[IBIS Ver]   4.1
[File name]   f29h85xzex.ibs
[File Rev]   1.0
[Date]   May 08,2024
[Source]   Cadence SpeedXP Suite XtractIM 18.0.4.05011.160686   004
[Notes]   One-Section RLC
[Disclaimer]   The model given below represents a 204-pin package.
[Copyright]
[Component] f29h85xzex
[Manufacturer] Texas Instruments
[Package]
|   Typ   Min   Max
R_pkg   0.159679576   0.033338   0.27914
L_pkg   3.09171E-09   1.037E-09   6.501E-09
C_pkg   4.79862E-13   3.114E-13   8.045E-13
[Pin]   Signal_name   model_name   R_pin   L_pin   C_pin
A10   GPIO30   BCF3355DSHYPBFZ_USF_7LM   1.45E-01   2.63E-09   3.38E-13
A11   GPIO83   BCF33100DSHYPBFZ_USF_7LM   0.14282   2.63E-09   3.32E-13
A12   GPIO81   BCF33100DSHYPBFZ_USF_7LM   0.14686   2.73E-09   3.47E-13
A13   GPIO77   BCF33100DSHYPBFZ_USF_7LM   0.14855   2.78E-09   4.09E-13
A14   GPIO72   BCF33100DSHYPBFZ_USF_7LM   0.15713   2.98E-09   4.19E-13
A15   GPIO69   BCF33100DSHYPBFZ_USF_7LM   0.14267   2.65E-09   4.90E-13
A2   GPIO13   BCF33100DSHYPBFZ_USF_7LM   1.43E-01   2.73E-09   4.52E-13
A3   GPIO12   BCF33100DSHYPBFZ_CORNER_USF_7LM   1.29E-01   2.21E-09   3.70E-13
A4   GPIO11   BCF33100DSHYPBFZ_USF_7LM   1.39E-01   2.63E-09   3.46E-13
A5   GPIO9   BCF3385DSHYPBFZ_USF_7LM   1.47E-01   2.75E-09   3.42E-13
A6   GPIO5   BCF33100DSHYPBFZ_USF_7LM   1.44E-01   2.67E-09   3.62E-13
A7   GPIO1   BCF33100DSHYPBFZ_USF_7LM   1.23E-01   2.07E-09   3.43E-13
A8   GPIO0   BCF33100DSHYPBFZ_USF_7LM   1.47E-01   2.73E-09   3.11E-13
A9   GPIO29   BQ33100HYPBFZ_PMB_5FS_LC_7LM   1.24E-01   2.04E-09   3.52E-13
B1   GPIO19   BCF33100DSHYPBFZ_USF_7LM   1.48E-01   2.78E-09   4.56E-13
B10   GPIO31   BCF33100DSHYPBFZ_USF_7LM   1.23E-01   2.03E-09   4.04E-13
B11   GPIO85   BCF33100DSHYPBFZ_USF_7LM   0.13246   2.41E-09   3.77E-13
B12   GPIO80   BCF33100DSHYPBFZ_USF_7LM   0.14179   2.59E-09   4.13E-13
B13   GPIO76   BCF33100DSHYPBFZ_USF_7LM   0.14931   2.86E-09   4.41E-13
B14   GPIO71   BCF33100DSHYPBFZ_USF_7LM   0.13499   2.41E-09   4.82E-13
B15   GPIO68   BCF33100DSHYPBFZ_CORNER_USF_7LM   0.12949   2.19E-09   4.03E-13
B16   GPIO67   BCF33100DSHYPBFZ_CORNER_USF_7LM   0.143   2.36E-09   4.11E-13
B2   GPIO17   BCF33100DSHYPBFZ_USF_7LM   1.60E-01   2.91E-09   4.98E-13
B3   GPIO14   BCF33100DSHYPBFZ_CORNER_USF_7LM   1.28E-01   2.08E-09   3.80E-13
B4   GPIO100   BCF33100DSHYPBFZ_USF_7LM   0.11781   2.04E-09   3.20E-13
B5   GPIO101   BCF33100DSHYPBFZ_USF_7LM   0.12464   2.10E-09   3.89E-13
B6   GPIO6   BCF3355DSHYPBFZ_USF_7LM   1.22E-01   2.04E-09   3.60E-13
B7   GPIO2   BCF33100DSHYPBFZ_USF_7LM   1.34E-01   2.44E-09   3.89E-13
B8   GPIO23   BQ33100HYPBFZ_PMB_5FS_LC_7LM   1.41E-01   2.62E-09   3.69E-13
B9   GPIO26   BCF33100DSHYPBFZ_USF_7LM   1.68E-01   3.36E-09   3.87E-13
C1   GPIO20   BCF33100DSHYPBFZ_USF_7LM   1.62E-01   3.26E-09   4.43E-13
C10   GPIO87   BCF33100DSHYPBFZ_USF_7LM   0.12649   2.12E-09   4.99E-13
C11   GPIO86   BCF33100DSHYPBFZ_USF_7LM   0.14552   2.67E-09   4.72E-13
C12   GPIO79   BCF33100DSHYPBFZ_USF_7LM   0.13263   2.32E-09   4.56E-13
C13   GPIO75   BCF33100DSHYPBFZ_USF_7LM   0.14056   2.47E-09   5.63E-13
C14   GPIO70   BCF3385DSHYPBFZ_CORNER_7LM   0.14317   2.50E-09   5.54E-13
C15   GPIO43   BCF33100DSHYPBFZ_CORNER_USF_7LM   0.15632   2.74E-09   4.12E-13
C16   GPIO42   BCPF335585DSHYPBFZ_USF_7LM   0.13495   2.31E-09   3.79E-13
C2   GPIO21   BCF33100DSHYPBFZ_USF_7LM   1.36E-01   2.50E-09   4.05E-13
C3   GPIO88   BCF33100DSHYPBFZ_USF_7LM   0.20709   4.07E-09   5.48E-13
C4   GPIO15   BQ33100HYPBFZ_PMB_5FS_LC_7LM   1.53E-01   2.53E-09   5.23E-13
C5   GPIO10   BQ33100HYPBFZ_PMB_5FS_LC_7LM   1.52E-01   2.77E-09   4.93E-13
C6   GPIO7   BCF33100DSHYPBFZ_USF_7LM   1.41E-01   2.49E-09   4.93E-13
C7   GPIO3   BCF33100DSHYPBFZ_USF_7LM   1.27E-01   2.12E-09   4.77E-13
C8   GPIO24   BCF33100DSHYPBFZ_USF_7LM   1.28E-01   2.12E-09   4.56E-13
C9   GPIO27   BCF33100DSHYPBFZ_USF_7LM   1.53E-01   2.81E-09   4.33E-13
D1   GPIO34   BCF33100DSHYPBFZ_USF_7LM   0.1782   3.51E-09   4.28E-13
D10   GPIO82   BCF33100DSHYPBFZ_USF_7LM   0.19065   3.73E-09   5.54E-13
D11   GPIO84   BCF33100DSHYPBFZ_USF_7LM   0.16159   2.88E-09   5.13E-13
D12   GPIO78   BCF33100DSHYPBFZ_USF_7LM   0.16009   3.23E-09   5.81E-13
D13   GPIO74   BCF33100DSHYPBFZ_USF_7LM   0.15949   3.19E-09   5.75E-13
D14   GPIO46   BCF33100DSHYPBFZ_USF_7LM   0.12327   1.89E-09   4.41E-13
D15   GPIO47   BCF33100DSHYPBFZ_USF_7LM   0.14294   2.62E-09   3.89E-13
D16   GPIO103   BCF33100DSHYPBFZ_USF_7LM   0.12938   2.13E-09   3.83E-13
D2   GPIO91   BCF33100DSHYPBFZ_USF_7LM   0.15495   2.87E-09   4.60E-13
D3   GPIO90   BCF33100DSHYPBFZ_USF_7LM   0.20167   3.98E-09   6.00E-13
D4   GPIO89   BCF33100DSHYPBFZ_USF_7LM   0.18558   3.67E-09   6.22E-13
D5   GPIO16   BCF33100DSHYPBFZ_USF_7LM   1.61E-01   2.51E-09   6.08E-13
D6   GPIO8   BCF33100DSHYPBFZ_USF_7LM   1.54E-01   2.98E-09   4.51E-13
D7   GPIO4   BCF33100DSHYPBFZ_USF_7LM   1.54E-01   2.71E-09   5.71E-13
D8   GPIO25   BCF33100DSHYPBFZ_USF_7LM   1.67E-01   3.27E-09   5.93E-13
D9   GPIO28   BCF33100DSHYPBFZ_USF_7LM   1.54E-01   2.72E-09   4.57E-13
E1   GPIO35   BCF33100DSHYPBFZ_USF_7LM   0.16952   3.23E-09   3.78E-13
E13   GPIO73   BCF33100DSHYPBFZ_USF_7LM   0.17483   3.52E-09   6.78E-13
E14   GPIO38   BCF33100DSHYPBFZ_USF_7LM   0.1436   2.49E-09   5.26E-13
E16   GPIO220,X1   BCPF335585DSHYPBFZ_USF_7LM   4.92E-02   1.43E-09   4.41E-13
E2   GPIO92   BCF3385DSHYPBFZ_USF_7LM   0.17361   3.35E-09   4.10E-13
E3   GPIO93   BCF33100DSHYPBFZ_USF_7LM   0.15008   2.68E-09   4.68E-13
E4   GPIO94   BCF33100DSHYPBFZ_USF_7LM   0.25902   5.43E-09   5.57E-13
E5   GPIO95   BCF33100DSHYPBFZ_USF_7LM   0.23782   5.10E-09   6.10E-13
F1   GPIO22   BQ33100HYPBFZ_PMB_5FS_LC_7LM   1.75E-01   3.52E-09   3.82E-13
F13   GPIO127   BCF33100DSHYPBFZ_USF_7LM   0.15682   3.16E-09   4.43E-13
F14   XRSn   BQ0491FS_3X2_USF_7LM   0.14283   2.45E-09   5.00E-13
F16   GPIO221,X2   BCPF335585DSHYPBFZ_USF_7LM   0.060019   1.35E-09   3.84E-13
F2   GPIO18   BQ33100HYPBFZ_PMB_5FS_LC_7LM   1.76E-01   3.43E-09   4.62E-13
F3   GPIO96   BCF33100DSHYPBFZ_USF_7LM   0.1653   3.12E-09   4.62E-13
F4   GPIO97   BCF33100DSHYPBFZ_USF_7LM   0.19143   3.93E-09   6.19E-13
F5   GPIO98   BCF33100DSHYPBFZ_USF_7LM   0.20928   4.00E-09   6.33E-13
G1   B11,GPIO235   BCF33100DSHYPBFZ_USF_7LM   1.58E-01   3.02E-09   3.27E-13
G13   GPIO66   BCF33100DSHYPBFZ_USF_7LM   0.17577   3.33E-09   5.59E-13
G14   GPIO44   BCF33100DSHYPBFZ_USF_7LM   0.14145   2.56E-09   4.00E-13
G15   GPIO45   BCF33100DSHYPBFZ_USF_7LM   0.13281   2.30E-09   3.62E-13
G16   GPIO32   BCF33100DSHYPBFZ_USF_7LM   1.40E-01   2.46E-09   3.27E-13
G2   B10,GPIO234   BCF33100DSHYPBFZ_USF_7LM   1.52E-01   2.90E-09   4.01E-13
G3   A10,GPIO228   BCF33100DSHYPBFZ_USF_7LM   1.56E-01   3.00E-09   4.95E-13
G4   A11,GPIO229   BCF33100DSHYPBFZ_USF_7LM   1.91E-01   3.93E-09   5.95E-13
G5   GPIO99   BCF33100DSHYPBFZ_USF_7LM   0.21088   4.13E-09   6.03E-13
H1   B9,GPIO233   BCF33100DSHYPBFZ_USF_7LM   1.62E-01   3.18E-09   4.59E-13
H13   GPIO62   BCF33100DSHYPBFZ_USF_7LM   0.17342   3.46E-09   5.40E-13
H14   GPIO63   BCF33100DSHYPBFZ_USF_7LM   0.13389   2.43E-09   4.22E-13
H15   GPIO64   BCF3385DSHYPBFZ_USF_7LM   0.13166   2.33E-09   3.69E-13
H16   GPIO65   BCF33100DSHYPBFZ_USF_7LM   0.14461   2.64E-09   3.20E-13
H2   B8,GPIO232   BCF33100DSHYPBFZ_USF_7LM   1.49E-01   2.88E-09   4.86E-13
H3   A9,GPIO227   BCF33100DSHYPBFZ_USF_7LM   1.52E-01   2.88E-09   4.89E-13
H4   A8,GPIO226   BCF33100DSHYPBFZ_USF_7LM   1.69E-01   3.47E-09   5.54E-13
H5   B7/E27,GPIO231   BCF33100DSHYPBFZ_USF_7LM   1.93E-01   3.96E-09   6.76E-13
J1   B13   ICF33SHYPB_LC_7LM   1.53E-01   3.05E-09   4.14E-13
J13   GPIO61   BCF33100DSHYPBFZ_USF_7LM   0.16898   3.19E-09   4.89E-13
J14   GPIO105   BCF33100DSHYPBFZ_USF_7LM   0.12843   2.17E-09   3.88E-13
J15   GPIO60   BCF33100DSHYPBFZ_USF_7LM   0.13505   2.37E-09   3.84E-13
J16   GPIO59   BCF3385DSHYPBFZ_USF_7LM   0.14954   2.75E-09   3.42E-13
J2   B12   ICF33SHYPB_LC_7LM   1.50E-01   2.94E-09   3.96E-13
J3   B17   ICF33SHYPB_LC_7LM   1.41E-01   2.71E-09   4.68E-13
J4   B16   ICF33SHYPB_LC_7LM   1.75E-01   3.37E-09   6.42E-13
J5   B6/E26,GPIO230   BCF33100DSHYPBFZ_USF_7LM   1.78E-01   3.63E-09   6.64E-13
K1   A13   ICF33SHYPB_LC_7LM   1.32E-01   2.41E-09   3.86E-13
K13   GPIO55   BCF33100DSHYPBFZ_USF_7LM   0.17624   3.49E-09   5.71E-13
K14   GPIO56   BCF33100DSHYPBFZ_USF_7LM   0.14006   2.55E-09   4.56E-13
K15   GPIO57   BCF33100DSHYPBFZ_USF_7LM   0.13532   2.34E-09   3.38E-13
K16   GPIO58   BCF33100DSHYPBFZ_USF_7LM   0.14501   2.61E-09   3.15E-13
K2   A12   ICF33SHYPB_LC_7LM   1.35E-01   2.48E-09   4.10E-13
K3   B5/D31   ICF33SHYPB_LC_7LM   1.61E-01   3.11E-09   4.97E-13
K4   B4/D30   ICF33SHYPB_LC_7LM   1.88E-01   3.80E-09   5.97E-13
K5   A7/E25,GPIO225   BCF33100DSHYPBFZ_USF_7LM   1.67E-01   3.46E-09   6.05E-13
L1   A5/D29   ICF33SHYPB_LC_7LM   1.53E-01   2.89E-09   3.51E-13
L14   GPIO52   BCF33100DSHYPBFZ_USF_7LM   0.16407   3.19E-09   4.14E-13
L15   GPIO53   BCF33100DSHYPBFZ_USF_7LM   0.14307   2.67E-09   3.58E-13
L16   GPIO54   BCF33100DSHYPBFZ_USF_7LM   0.15266   2.85E-09   3.17E-13
L2   A4/D28   ICF33SHYPB_LC_7LM   1.51E-01   2.87E-09   3.95E-13
L3   B3/D27   ICF33SHYPB_LC_7LM   1.10E-01   2.16E-09   4.65E-13
L4   B2/D26   ICF33SHYPB_LC_7LM   1.19E-01   2.52E-09   4.84E-13
L5   A6/E24,GPIO224   BCF33100DSHYPBFZ_USF_7LM   1.86E-01   4.00E-09   5.82E-13
M1   A2/D24   ICF33SHYPB_LC_7LM   1.82E-01   3.69E-09   4.08E-13
M12   FLT3   NC   1.67E-01   3.57E-09   5.24E-13
M13   GPIO51   BCF33100DSHYPBFZ_USF_7LM   0.14778   2.76E-09   5.58E-13
M14   GPIO50   BCF33100DSHYPBFZ_USF_7LM   0.12773   2.25E-09   4.32E-13
M15   GPIO49   BCF33100DSHYPBFZ_USF_7LM   0.1387   2.54E-09   3.84E-13
M16   GPIO219/ERRORSTS   BCF33100DSHYPBFZ_CORNER_USF_7LM   1.51E-01   2.78E-09   3.19E-13
M2   A3/D25   ICF33SHYPB_LC_7LM   1.49E-01   2.79E-09   3.98E-13
M3   A14/B14/C14/D14/E14   ICF33SHYPB_LC_7LM   1.86E-01   3.63E-09   4.91E-13
M4   A15/B15/C15/D15/E15   ICF33SHYPB_LC_7LM   1.93E-01   4.05E-09   5.10E-13
M5   C3/E31   ICF33SHYPB_LC_7LM   1.86E-01   3.93E-09   7.70E-13
M6   D13   ICF33SHYPB_LC_7LM   1.78E-01   3.72E-09   5.83E-13
M7   D12   ICF33SHYPB_LC_7LM   2.03E-01   4.33E-09   6.13E-13
M8   C6,GPIO236   BCF33100DSHYPBFZ_USF_7LM   1.95E-01   4.01E-09   6.43E-13
M9   C7,GPIO237   BCF33100DSHYPBFZ_USF_7LM   1.88E-01   3.84E-09   5.77E-13
N1   VREFLOAB   NC   0.066124   1.95E-09   4.25E-13
N10   D4/B28,GPIO240   BCF33100DSHYPBFZ_USF_7LM   1.99E-01   4.23E-09   6.21E-13
N11   D5/B29,GPIO241   BCF33100DSHYPBFZ_USF_7LM   2.06E-01   4.64E-09   6.26E-13
N12   C8,GPIO238   BCF33100DSHYPBFZ_USF_7LM   2.73E-01   6.23E-09   7.41E-13
N13   E7/A31,GPIO249   BCF33100DSHYPBFZ_USF_7LM   2.30E-01   4.92E-09   7.59E-13
N14   GPIO36   BCF33100DSHYPBFZ_7LM   0.19862   3.66E-09   7.25E-13
N15   GPIO41   BCF33100DSHYPBFZ_CORNER_USF_7LM   0.14183   2.56E-09   3.74E-13
N16   GPIO48   BCF33100DSHYPBFZ_USF_7LM   0.1406   2.41E-09   3.31E-13
N2   VREFHIAB   NC   0.055738   1.97E-09   4.95E-13
N3   B1/C27   ICF33SHYPB_LC_7LM   1.75E-01   3.32E-09   4.83E-13
N4   C2/E30   ICF33SHYPB_LC_7LM   1.76E-01   3.65E-09   7.61E-13
N5   C5   ICF33SHYPB_LC_7LM   9.28E-02   1.96E-09   7.28E-13
N6   D10   ICF33SHYPB_LC_7LM   1.77E-01   3.51E-09   5.14E-13
N7   C16   ICF33SHYPB_LC_7LM   1.71E-01   3.49E-09   5.62E-13
N8   C10   ICF33SHYPB_LC_7LM   1.92E-01   4.15E-09   6.12E-13
N9   E13   ICF33SHYPB_LC_7LM   2.66E-01   6.15E-09   7.62E-13
P1   A1/C25   ICF33SHYPB_LC_7LM   1.71E-01   3.07E-09   3.92E-13
P10   E16   ICF33SHYPB_LC_7LM   1.79E-01   3.54E-09   5.07E-13
P11   E4/A28,GPIO246   BCF33100DSHYPBFZ_USF_7LM   1.88E-01   3.79E-09   5.25E-13
P12   C9,GPIO239   BCF33100DSHYPBFZ_USF_7LM   2.26E-01   5.03E-09   6.33E-13
P13   E6/A30,GPIO248   BCF33100DSHYPBFZ_USF_7LM   1.97E-01   3.93E-09   7.36E-13
P14   GPIO33   BCF33100DSHYPBFZ_7LM   0.18528   3.48E-09   5.63E-13
P15   GPIO39   BCF33100DSHYPBFZ_7LM   0.2243   4.33E-09   4.91E-13
P16   GPIO40   BCF33100DSHYPBFZ_7LM   0.16459   3.13E-09   4.64E-13
P2   B0/C26/VDAC   ICF33SHYPB_LC_7LM   1.78E-01   3.30E-09   4.66E-13
P3   E0/A24/DACC_OUT   ICF33SHYPB_LC_7LM   1.38E-01   2.43E-09   5.71E-13
P4   E1/A25   ICF33SHYPB_LC_7LM   1.35E-01   2.38E-09   6.11E-13
P5   C4   ICF33SHYPB_LC_7LM   8.63E-02   1.54E-09   7.18E-13
P6   D11   ICF33SHYPB_LC_7LM   2.14E-01   4.78E-09   6.22E-13
P7   C17   ICF33SHYPB_LC_7LM   2.12E-01   4.70E-09   6.01E-13
P8   C11   ICF33SHYPB_LC_7LM   1.96E-01   4.14E-09   5.94E-13
P9   E12   ICF33SHYPB_LC_7LM   2.79E-01   6.50E-09   8.05E-13
R1   A0/C24/DACA_OUT   ICF33SHYPB_LC_7LM   1.91E-01   3.62E-09   3.84E-13
R10   E10   ICF33SHYPB_LC_7LM   2.15E-01   4.60E-09   5.82E-13
R11   E5/A29,GPIO247   BCF33100DSHYPBFZ_USF_7LM   1.67E-01   3.21E-09   5.05E-13
R12   D7/B31,GPIO243   BCF33100DSHYPBFZ_USF_7LM   2.16E-01   4.58E-09   5.28E-13
R13   D8/C28,GPIO244   BCF33100DSHYPBFZ_USF_7LM   2.32E-01   4.96E-09   5.66E-13
R14   GPIO223/TDO   BCPF335585DSHYPBFZ_USF_7LM   0.20498   4.09E-09   5.17E-13
R15   TCK   IQ0442FS_40P60P_3X2_USF_7LM   0.20021   3.98E-09   5.32E-13
R16   GPIO37   BCF33100DSHYPBFZ_7LM   0.20499   4.11E-09   4.81E-13
R2   C0/E28   ICF33SHYPB_LC_7LM   1.62E-01   2.97E-09   4.04E-13
R3   D0/B24   ICF33SHYPB_LC_7LM   1.52E-01   2.77E-09   5.12E-13
R4   VREFHICDE   NC   0.033338   1.04E-09   3.47E-13
R5   D2/B26   ICF33SHYPB_LC_7LM   1.38E-01   2.57E-09   3.55E-13
R6   D3/B27   ICF33SHYPB_LC_7LM   1.30E-01   2.35E-09   3.54E-13
R7   D16   ICF33SHYPB_LC_7LM   1.38E-01   2.57E-09   3.57E-13
R8   C12   ICF33SHYPB_LC_7LM   1.31E-01   2.29E-09   3.98E-13
R9   E11   ICF33SHYPB_LC_7LM   1.80E-01   3.64E-09   5.59E-13
T10   E8/C30   ICF33SHYPB_LC_7LM   1.78E-01   3.62E-09   4.04E-13
T11   E17   ICF33SHYPB_LC_7LM   2.17E-01   4.54E-09   5.56E-13
T12   D6/B30,GPIO242   BCF33100DSHYPBFZ_USF_7LM   1.78E-01   3.46E-09   4.08E-13
T13   D9/C29,GPIO245   BCF33100DSHYPBFZ_USF_7LM   1.79E-01   3.36E-09   5.62E-13
T14   GPIO222/TDI   BCF33100DSHYPBFZ_USF_7LM   0.22961   4.78E-09   5.48E-13
T15   TMS   BCF3355DSHYPBFZ_TMS_USF_7LM   0.20987   4.29E-09   5.16E-13
T2   C1/E29   ICF33SHYPB_LC_7LM   1.72E-01   3.35E-09   4.89E-13
T3   D1/B25   ICF33SHYPB_LC_7LM   1.41E-01   2.46E-09   5.13E-13
T4   VREFLOCDE   NC   0.058365   1.77E-09   3.21E-13
T5   E2/A26   ICF33SHYPB_LC_7LM   1.37E-01   2.50E-09   3.26E-13
T6   E3/A27   ICF33SHYPB_LC_7LM   1.26E-01   2.16E-09   3.18E-13
T7   D17   ICF33SHYPB_LC_7LM   1.41E-01   2.60E-09   3.34E-13
T8   C13   ICF33SHYPB_LC_7LM   1.42E-01   2.59E-09   3.52E-13
T9   E9/C31   ICF33SHYPB_LC_7LM   1.55E-01   2.93E-09   3.80E-13
| End of package information
|   Component BCF33100DSHYPBFZ_7LM
[Component]   BCF33100DSHYPBFZ_7LM
[Manufacturer]  IO Methodology Inc.
[Package]
|   typ   min   max
R_pkg   0   0   0
L_pkg   0   0   0
C_pkg   0   0   0
[Pin]   signal_name  model_name   R_pin   L_pin   C_pin
VSS   VSS   GND
VDDS   VDDS   POWER
PAD   PAD   BCF33100DSHYPBFZ_7LM
[Model Selector] BCF33100DSHYPBFZ_7LM
WK_PU_ON_3P3  Cell operated at 3.3(nom)
|WK_PU_ON_3P3; WEAK_PULLUP_ON
WK_PD_ON_3P3  Cell operated at 3.3(nom)
|WK_PD_ON_3P3; WEAK_PULLDOWN_ON
DRIVER_MODE_3P3  Cell operated at 3.3(nom)
|DRIVER_MODE_3P3
RECEIVER_MODE_3P3  Cell operated at 3.3(nom)
|   Component BCF33100DSHYPBFZ_USF_7LM
[Component]   BCF33100DSHYPBFZ_USF_7LM
[Manufacturer]  Texas Instruments
[Package]
| variable   typ   min   max
R_pkg   0.0   0.0   0.0
L_pkg   0.0H   0.0H   0.0H
C_pkg   0.0F   0.0F   0.0F
[Pin]  signal_name   model_name   R_pin   L_pin   C_pin
PAD   PAD   BCF33100_USF_7LM_IO_3.3V   0   0   0
VDDS   VDDS   Power   0   0   0
VSS   VSS   Gnd   0   0   0
[Model Selector] BCF33100DSHYPBFZ_USF_7LM
BCF33100_USF_7LM_IO_3.3V I/O model with 3.3V supply
|   Component BCF33100DSHYPBFZ_CORNER_USF_7LM
[Component]   BCF33100DSHYPBFZ_CORNER_USF_7LM
[Manufacturer]  Texas Instruments
[Package]
| variable   typ   min   max
R_pkg   0.0   0.0   0.0
L_pkg   0.0H   0.0H   0.0H
C_pkg   0.0F   0.0F   0.0F
[Pin]  signal_name   model_name   R_pin   L_pin   C_pin
PAD   PAD   BCF33100_CORNER_7LM_IO_3.3V   0   0   0
VDDS   VDDS   Power   0   0   0
VSS   VSS   Gnd   0   0   0
[Model Selector] BCF33100DSHYPBFZ_CORNER_USF_7LM
BCF33100_CORNER_7LM_IO_3.3V  I/O model with 3.3V supply
|   Component BCF3355DSHYPBFZ_TMS_USF_7LM
[Component]   BCF3355DSHYPBFZ_TMS_USF_7LM
[Manufacturer]  Texas Instruments
[Package]
| variable   typ   min   max
R_pkg   0.0   0.0   0.0
L_pkg   0.0H   0.0H   0.0H
C_pkg   0.0F   0.0F   0.0F
[Pin]  signal_name   model_name   R_pin   L_pin   C_pin
PAD   PAD   BCF3355_TMS_7LM_IO_3.3V   0   0   0
VDDS   VDDS   Power   0   0   0
VSS   VSS   Gnd   0   0   0
[Model Selector] BCF3355DSHYPBFZ_TMS_USF_7LM
BCF3355_TMS_7LM_IO_3.3V I/O model with 3.3V supply
|   Component IQ0442FS_40P60P_3X2_USF_7LM
[Component]   IQ0442FS_40P60P_3X2_USF_7LM
[Manufacturer]  Texas Instruments
[Package]
| variable   typ   min   max
R_pkg   0.0   0.0   0.0
L_pkg   0.0H   0.0H   0.0H
C_pkg   0.0F   0.0F   0.0F
[Pin]  signal_name   model_name   R_pin   L_pin   C_pin
PAD   PAD   IQRX_3.3V   0   0   0
VDDS   VDDS   Power   0   0   0
VSS   VSS   Gnd   0   0   0
[Model Selector] IQ0442FS_40P60P_3X2_USF_7LM
IQRX_3.3V I/O model with 3.3V supply
|   Component BCF3355DSHYPBFZ_USF_7LM
[Component]   BCF3355DSHYPBFZ_USF_7LM
[Manufacturer]  Texas Instruments
[Package]
| variable   typ   min   max
R_pkg   0.0   0.0   0.0
L_pkg   0.0H   0.0H   0.0H
C_pkg   0.0F   0.0F   0.0F
[Pin]  signal_name   model_name   R_pin   L_pin   C_pin
PAD   PAD   BCF3355_USF_7LM_IO_3.3V   0   0   0
VDDS   VDDS   Power   0   0   0
VSS   VSS   Gnd   0   0   0
[Model Selector] BCF3355DSHYPBFZ_USF_7LM
BCF3355_USF_7LM_IO_3.3V I/O model with 3.3V supply
|   Component BCF3385DSHYPBFZ_CORNER_7LM
[Component]   BCF3385DSHYPBFZ_CORNER_7LM
[Manufacturer]  IO Methodology Inc.
[Package]
|   typ   min   max
R_pkg   0   0   0
L_pkg   0   0   0
C_pkg   0   0   0
[Pin]   signal_name  model_name   R_pin   L_pin   C_pin
VSS   VSS   GND
VDDS   VDDS   POWER
PAD   PAD   BCF3385DSHYPBFZ_CORNER_7LM
[Model Selector] BCF3385DSHYPBFZ_CORNER_7LM
WK_PU_ON_3P3_BCF3385DSHYPBFZ_CORNER_7LM  Cell operated at 3.3(nom)
|WK_PU_ON_3P3; WEAK_PULLUP_ON
WK_PD_ON_3P3_BCF3385DSHYPBFZ_CORNER_7LM  Cell operated at 3.3(nom)
|WK_PD_ON_3P3; WEAK_PULLDOWN_ON
DRIVER_MODE_3P3_BCF3385_CORNER_7LM Cell operated at 3.3(nom)
|DRIVER_MODE_3P3
RECEIVER_MODE_3P3_BCF3385_CORNER_7LM  Cell operated at 3.3(nom)
|   Component BCF3385DSHYPBFZ_USF_7LM
[Component]   BCF3385DSHYPBFZ_USF_7LM
[Manufacturer]  Texas Instruments
[Package]
| variable   typ   min   max
R_pkg   0.0   0.0   0.0
L_pkg   0.0H   0.0H   0.0H
C_pkg   0.0F   0.0F   0.0F
[Pin]  signal_name   model_name   R_pin   L_pin   C_pin
PAD   PAD   BCF3385_USF_7LM_IO_3.3V   0   0   0
VDDS   VDDS   Power   0   0   0
VSS   VSS   Gnd   0   0   0
[Model Selector] BCF3385DSHYPBFZ_USF_7LM
BCF3385_USF_7LM_IO_3.3V I/O model with 3.3V supply
|   Component BCPF335585DSHYPBFZ_USF_7LM
[Component]   BCPF335585DSHYPBFZ_USF_7LM
[Manufacturer]  Texas Instruments
[Package]
| variable   typ   min   max
R_pkg   0.0   0.0   0.0
L_pkg   0.0H   0.0H   0.0H
C_pkg   0.0F   0.0F   0.0F
[Pin]  signal_name   model_name   R_pin   L_pin   C_pin
PAD   PAD   BCPF335585DSHYPBFZ_USF_7LM   0   0   0
VDDS   VDDS   Power   0   0   0
VSS   VSS   Gnd   0   0   0
[Model Selector]   BCPF335585DSHYPBFZ_USF_7LM
BCPF335585_7LM_IO_DS0_3.3V   I/O model DS 0 with 3.3V supply
BCPF335585_7LM_IO_DS1_3.3V   I/O model DS 1 with 3.3V supply
|   Component BQ0491FS_3X2_USF_7LM
[Component]   BQ0491FS_3X2_USF_7LM
[Manufacturer]  Texas Instruments
[Package]
| variable   typ   min   max
R_pkg   0.0   0.0   0.0
L_pkg   0.0H   0.0H   0.0H
C_pkg   0.0F   0.0F   0.0F
[Pin]  signal_name   model_name   R_pin   L_pin   C_pin
PAD   PAD   BQ0491FS_3X2_USF_7LM   0   0   0
VDDS   VDDS   Power   0   0   0
VSS   VSS   Gnd   0   0   0
[Model Selector]   BQ0491FS_3X2_USF_7LM
BQ0491_3X2_USF_7LM_IO_15p_3p3   I/O open drain model with C_fixture 15pF for 3.3V supply
BQ0491_3X2_USF_7LM_IO_50p_3p3   I/O open drain model with C_fixture 50pF for 3.3V supply
BQ0491_3X2_USF_7LM_IO_100p_3p3   I/O open drain model with C_fixture 100pF for 3.3V supply
BQ0491_3X2_USF_7LM_IO_150p_3p3   I/O open drain model with C_fixture 150pF for 3.3V supply
|   Component BQ33100HYPBFZ_PMB_5FS_LC_7LM
[Component]   BQ33100HYPBFZ_PMB_5FS_LC
[Manufacturer]  Texas Instruments
[Package]
| variable   typ   min   max
R_pkg   0.0   0.0   0.0
L_pkg   0.0H   0.0H   0.0H
C_pkg   0.0F   0.0F   0.0F
[Pin]  signal_name   model_name   R_pin   L_pin   C_pin
Pin1   PAD   BQ33100HYPBFZ_PMB_5FS_LC_7LM   0   0   0
Pin2   VDDS   Power   0   0   0
Pin3   VSS   Gnd   0   0   0
[Model Selector]   BQ33100HYPBFZ_PMB_5FS_LC_7LM
BQ33_PMB_IO_M0_D0   I/O model with Mode = 0 and Drive = 0
BQ33_PMB_IO_M0_D1   I/O model with Mode = 0 and Drive = 1
BQ33_PMB_IO_M1_D0   I/O model with Mode = 1 and Drive = 0
BQ33_PMB_IO_M1_D1   I/O model with Mode = 1 and Drive = 1
|   Component IQ0440FS_VREGENZ_PU_7LM
[Component]   IQ0440FS_VREGENZ_PU_7LM
[Manufacturer]  Texas Instruments
[Package]
|   typ   min   max
R_pkg   0   0   0
L_pkg   0   0   0
C_pkg   0   0   0
[Pin]   signal_name  model_name   R_pin   L_pin   C_pin
VSS   VSS   GND
VDDS   VDDS   POWER
PAD   PAD   IQ0440FS_VREGENZ_PU_7LM
[Model Selector] IQ0440FS_VREGENZ_PU_7LM
WK_PD_ON_3P3_IQ0440FS_VREGENZ_PU_7LM Cell operated at 3.3(nom)
|WK_PD_ON_3P3; WEAK_PULLDOWN_ON
RECEIVER_MODE_3P3_IQ0440FS_VREGENZ  Cell operated at 3.3(nom)
|   Component ICF33SHYPB_LC_7LM
[Component]   ICF33SHYPB_LC_7LM
[Manufacturer]   Texas Instruments
[Package]
|  variable   typ   min   max
R_pkg   0   0   0
L_pkg   0   0   0
C_pkg   0   0   0
[Pin]   signal_name   model_name   R_pin   L_pin   C_pin
VSS   VSS   GND
VDDS   VDDS   POWER
PAD   PAD   ICF33SHYPB_LC_7LM
[Model Selector] ICF33SHYPB_LC_7LM
RECEIVER_MODE_3P3_ICF_7LM  Cell operated at 3.3(nom)
|RECEIVER_MODE_3P3_ICF_7LM; RECEIVER_MODE
WK_PU_ON_3P3_ICF_7LM  Cell operated at 3.3(nom)
|WK_PU_ON_3P3_ICF_7LM; WEAK_PULLUP_ON
WK_PD_ON_3P3_ICF_7LM  Cell operated at 3.3(nom)
| Models and submodels in the file (29): WK_PU_ON_3P3 (Input), WK_PD_ON_3P3 (Input), DRIVER_MODE_3P3 (I/O), RECEIVER_MODE_3P3 (Input), BCF33100_USF_7LM_IO_3.3V (I/O), BCF33100_CORNER_7LM_IO_3.3V (I/O), BCF3355_TMS_7LM_IO_3.3V (I/O), IQRX_3.3V (Input), BCF3355_USF_7LM_IO_3.3V (I/O), WK_PU_ON_3P3_BCF3385DSHYPBFZ_CORNER_7LM (Input), WK_PD_ON_3P3_BCF3385DSHYPBFZ_CORNER_7LM (Input), DRIVER_MODE_3P3_BCF3385_CORNER_7LM (I/O), RECEIVER_MODE_3P3_BCF3385_CORNER_7LM (Input), BCF3385_USF_7LM_IO_3.3V (I/O), BCPF335585_7LM_IO_DS0_3.3V (I/O), BCPF335585_7LM_IO_DS1_3.3V (I/O), BQ0491_3X2_USF_7LM_IO_15p_3p3 (I/O_open_drain), BQ0491_3X2_USF_7LM_IO_50p_3p3 (I/O_open_drain), BQ0491_3X2_USF_7LM_IO_100p_3p3 (I/O_open_drain), BQ0491_3X2_USF_7LM_IO_150p_3p3 (I/O_open_drain), BQ33_PMB_IO_M0_D0 (I/O), BQ33_PMB_IO_M0_D1 (I/O), BQ33_PMB_IO_M1_D0 (I/O), BQ33_PMB_IO_M1_D1 (I/O), WK_PD_ON_3P3_IQ0440FS_VREGENZ_PU_7LM (Input), RECEIVER_MODE_3P3_IQ0440FS_VREGENZ (Input), RECEIVER_MODE_3P3_ICF_7LM (Input), WK_PU_ON_3P3_ICF_7LM (Input), WK_PD_ON_3P3_ICF_7LM (Input)
